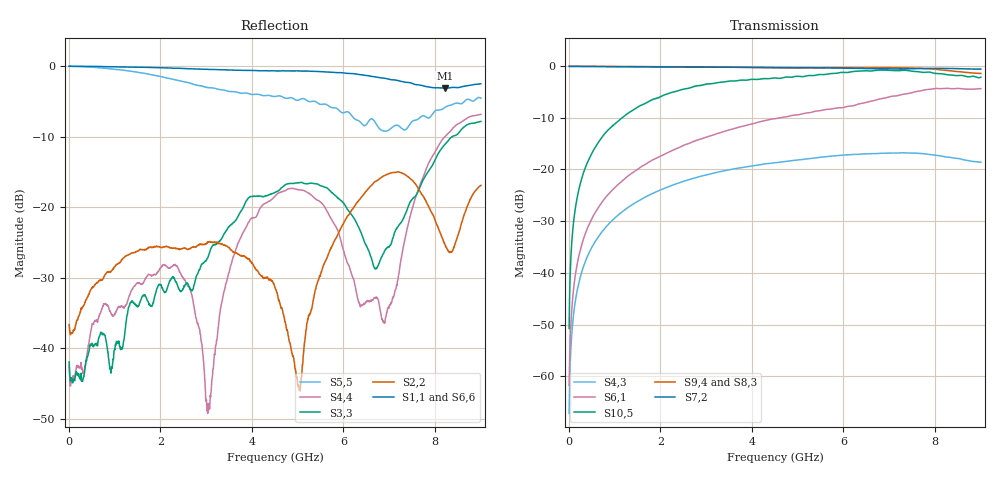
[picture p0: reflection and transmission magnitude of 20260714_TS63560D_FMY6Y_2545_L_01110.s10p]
# GHz S DB R 50
! CMT, SN0916, 25263762, 26.7.0
! Date: 15.07.2026 13:40:29
! Data: Format
! Freq S1.1:dB/Ang S1.2:dB/Ang S1.3:dB/Ang S1.4:dB/Ang S1.5:dB/Ang S1.6:dB/Ang S1.7:dB/Ang S1.8:dB/Ang S1.9:dB/Ang S1.10:dB/Ang
!  S2.1:dB/Ang S2.2:dB/Ang S2.3:dB/Ang S2.4:dB/Ang S2.5:dB/Ang S2.6:dB/Ang S2.7:dB/Ang S2.8:dB/Ang S2.9:dB/Ang S2.10:dB/Ang
!  S3.1:dB/Ang S3.2:dB/Ang S3.3:dB/Ang S3.4:dB/Ang S3.5:dB/Ang S3.6:dB/Ang S3.7:dB/Ang S3.8:dB/Ang S3.9:dB/Ang S3.10:dB/Ang
!  S4.1:dB/Ang S4.2:dB/Ang S4.3:dB/Ang S4.4:dB/Ang S4.5:dB/Ang S4.6:dB/Ang S4.7:dB/Ang S4.8:dB/Ang S4.9:dB/Ang S4.10:dB/Ang
!  S5.1:dB/Ang S5.2:dB/Ang S5.3:dB/Ang S5.4:dB/Ang S5.5:dB/Ang S5.6:dB/Ang S5.7:dB/Ang S5.8:dB/Ang S5.9:dB/Ang S5.10:dB/Ang
!  S6.1:dB/Ang S6.2:dB/Ang S6.3:dB/Ang S6.4:dB/Ang S6.5:dB/Ang S6.6:dB/Ang S6.7:dB/Ang S6.8:dB/Ang S6.9:dB/Ang S6.10:dB/Ang
!  S7.1:dB/Ang S7.2:dB/Ang S7.3:dB/Ang S7.4:dB/Ang S7.5:dB/Ang S7.6:dB/Ang S7.7:dB/Ang S7.8:dB/Ang S7.9:dB/Ang S7.10:dB/Ang
!  S8.1:dB/Ang S8.2:dB/Ang S8.3:dB/Ang S8.4:dB/Ang S8.5:dB/Ang S8.6:dB/Ang S8.7:dB/Ang S8.8:dB/Ang S8.9:dB/Ang S8.10:dB/Ang
!  S9.1:dB/Ang S9.2:dB/Ang S9.3:dB/Ang S9.4:dB/Ang S9.5:dB/Ang S9.6:dB/Ang S9.7:dB/Ang S9.8:dB/Ang S9.9:dB/Ang S9.10:dB/Ang
!  S10.1:dB/Ang S10.2:dB/Ang S10.3:dB/Ang S10.4:dB/Ang S10.5:dB/Ang S10.6:dB/Ang S10.7:dB/Ang S10.8:dB/Ang S10.9:dB/Ang S10.10:dB/Ang
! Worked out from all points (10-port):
!   2001 points, 10 MHz to 9 GHz, reference 50 ohm
!   strongest paths, dB at 10 MHz, 2.257 GHz, 4.505 GHz, 6.753 GHz, 9 GHz:
!     S7,2: -0.1, -0.2, -0.3, -0.6, -0.6
!     S9,4: -0.1, -0.2, -0.4, -0.4, -1.5
!     S8,3: -0.1, -0.2, -0.4, -0.4, -1.3
!     S10,5: -50.7, -5.1, -2.4, -0.8, -2.2
!     S6,1: -61.7, -16.4, -10.2, -6.5, -4.4
!     S4,3: -67.1, -23.1, -18.7, -16.9, -18.6
!   lowest |S11| = -3.1 dB at 8.213 GHz (marker M1), VSWR 5.62, Z = 11 - j23.8 ohm
!   |S11| at or under -10 dB: nowhere
